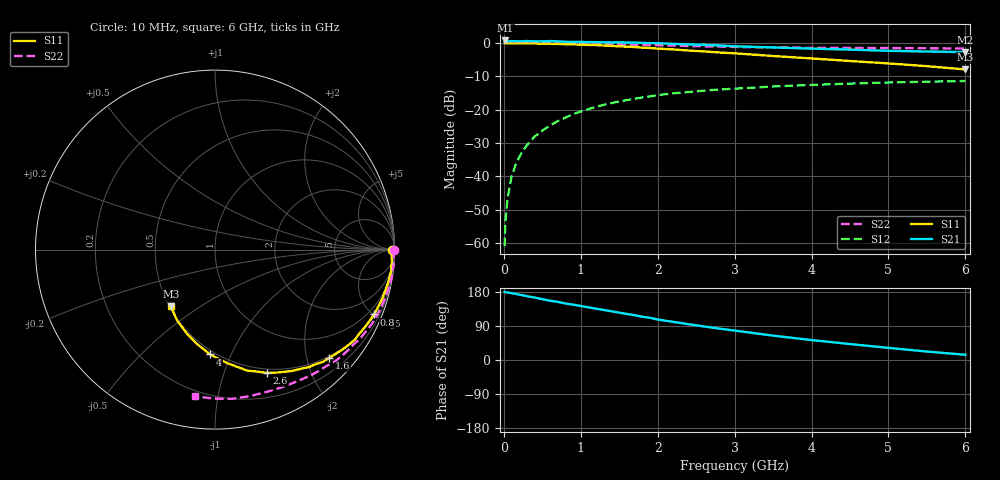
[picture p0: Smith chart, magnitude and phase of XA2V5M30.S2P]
! SIEMENS Discrete & RF Semiconductors
! BFY180
! Si NPN RF Bipolar Junction Transistor in MICRO-X
! VCE = 2.5 V  IC = 0.3 mA
! Common Emitter S-Parameters:  May  1997
# GHz  S  MA  R  50
!  f  S11  S21  S12  S22
! GHz  MAG  ANG  MAG  ANG  MAG  ANG  MAG  ANG
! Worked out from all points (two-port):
!   36 points, 10 MHz to 6 GHz, reference 50 ohm
!   highest |S21| = 0.73 dB at 20 MHz (marker M1); lowest = -2.8 dB at 6 GHz (marker M2)
!   |S21| within 3 dB of the highest: start of sweep to 4.853 GHz
!   lowest |S11| = -8.0 dB at 6 GHz (marker M3), VSWR 2.33, Z = 25.4 - j19.1 ohm
!   |S11| at or under -10 dB: nowhere
!   |S22| runs from -1.7 to 0.0 dB; largest |S21 - S12| = 1.1
!   S11 on the Smith chart (normalised r, x): 10 MHz: open; 800 MHz: 0.59, -5.03; 1.6 GHz: 0.46, -2.42; 2.6 GHz: 0.45, -1.41; 4 GHz: 0.47, -0.84; 6 GHz: 0.51, -0.38
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0.01  0.987 -0.2  1.051 179.9  0.0009 90.6  0.9984 -0.1
0.02  0.9917 -0.7  1.088 179.1  0.0021 83.9  0.9997 -0.4
0.05  0.9855 -1.4  1.054 178.1  0.0048 85.5  0.999 -1.1
0.1  0.9857 -2.5  1.061 176.3  0.0099 88.2  0.9955 -2.1
0.15  0.989 -4.3  1.06 174.6  0.0146 87.6  0.9999 -3.2
0.25  0.9891 -7.0  1.059 170.7  0.0246 85.3  0.9991 -5.3
0.4  0.9817 -11.0  1.053 164.8  0.0395 81.4  0.9972 -8.4
0.5  0.9749 -14.0  1.058 160.5  0.0486 78.4  0.9944 -10.5
0.6  0.97 -16.9  1.066 156.4  0.0578 76.3  0.9905 -12.6
0.7  0.9624 -19.6  1.055 153.5  0.0673 73.6  0.9884 -14.7
0.8  0.9566 -22.2  1.039 149.1  0.076 71.5  0.9839 -16.7
1.1  0.9307 -30.1  1.03 138.9  0.1019 64.8  0.9717 -22.7
1.6  0.877 -43.6  1.015 121.4  0.1392 53.9  0.9439 -32.6
1.9  0.839 -51.2  0.994 111.3  0.158 48.0  0.9266 -38.0
2  0.8218 -53.7  0.991 106.9  0.1651 46.3  0.9232 -39.7
2.2  0.7988 -57.9  0.967 100.7  0.1752 42.4  0.9125 -43.3
2.6  0.7462 -67.1  0.934 88.5  0.1924 35.9  0.889 -49.6
3.5  0.6363 -83.8  0.855 64.3  0.2223 23.5  0.8559 -62.6
4  0.5849 -92.6  0.821 52.6  0.2345 17.3  0.8443 -69.6
4.5  0.5354 -100.8  0.793 42.1  0.2456 11.8  0.8394 -76.4
5.5  0.4481 -118.1  0.743 22.3  0.2622 1.1  0.8305 -90.6
6  0.4001 -128.0  0.727 13.8  0.2686 -4.4  0.8238 -97.7
